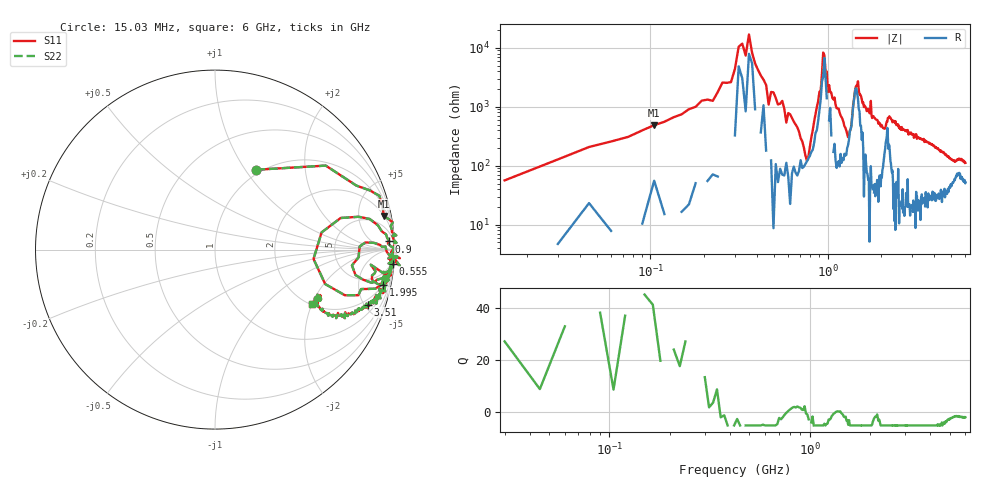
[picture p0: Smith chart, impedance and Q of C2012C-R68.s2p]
!	Network	Analyzer	HP8753E.07.74:	Oct	30	2002	Serial	No.	JP38451487
!	Hewlett-Packard
!	28	Aug	2009	12:47:42
!	Frequency	S11	S21	S12	S22
#	HZ	S	RI	R	50
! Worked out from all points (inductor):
!   400 points, 15.03 MHz to 6 GHz, reference 50 ohm
!   read as one part in series: L = 663 nH near 45.03 MHz
!   highest Q = 32.8 at 105 MHz (marker M1), where L = 735 nH
!   self-resonance near 345 MHz
!   S11 on the Smith chart (normalised r, x): 15.03 MHz: 0.95, +1.13; 555 MHz: 3, -25; 900 MHz: 19, +31; 1.995 GHz: 1.91, -9.24; 3.51 GHz: 1.55, -5.29; 6 GHz: 2.04, -1.98
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1.502992e7  0.231 0.445  0.769 -0.445  0.769 -0.445  0.231 0.445
4.502978e7  0.787 0.357  0.213 -0.357  0.213 -0.357  0.787 0.357
1.050295e8  0.94 0.187  0.0601 -0.187  0.0601 -0.187  0.94 0.187
2.850286e8  1.01 0.0383  -0.00506 -0.0383  -0.00506 -0.0383  1.01 0.0383
3.150284e8  0.995 0.00842  0.00452 -0.00842  0.00452 -0.00842  0.995 0.00842
3.450283e8  0.998 0.0134  0.00171 -0.0134  0.00171 -0.0134  0.998 0.0134
3.600282e8  0.997 -0.00522  0.00281 0.00522  0.00281 0.00522  0.997 -0.00522
4.650277e8  1.03 -0.0912  -0.0258 0.0912  -0.0258 0.0912  1.03 -0.0912
5.550272e8  0.989 -0.0781  0.0106 0.0781  0.0106 0.0781  0.989 -0.0781
7.650262e8  0.549 -0.0521  0.451 0.0521  0.451 0.0521  0.549 -0.0521
9.000255e8  0.971 0.0457  0.0289 -0.0457  0.0289 -0.0457  0.971 0.0457
9.450253e8  0.995 0.011  0.00482 -0.011  0.00482 -0.011  0.995 0.011
1.020025e9  0.988 -0.0405  0.0123 0.0405  0.0123 0.0405  0.988 -0.0405
1.305023e9  0.783 -0.142  0.217 0.142  0.217 0.142  0.783 -0.142
1.485023e9  0.981 -0.0306  0.0194 0.0306  0.0194 0.0306  0.981 -0.0306
1.99502e9  0.938 -0.197  0.0617 0.197  0.0617 0.197  0.938 -0.197
2.01002e9  0.935 -0.184  0.0645 0.184  0.0645 0.184  0.935 -0.184
3.015015e9  0.923 -0.271  0.0769 0.271  0.0769 0.271  0.923 -0.271
3.510012e9  0.852 -0.307  0.148 0.307  0.148 0.307  0.852 -0.307
4.00501e9  0.791 -0.348  0.209 0.348  0.209 0.348  0.791 -0.348
5.010005e9  0.592 -0.331  0.408 0.331  0.408 0.331  0.592 -0.331
6e9  0.538 -0.301  0.462 0.301  0.462 0.301  0.538 -0.301
